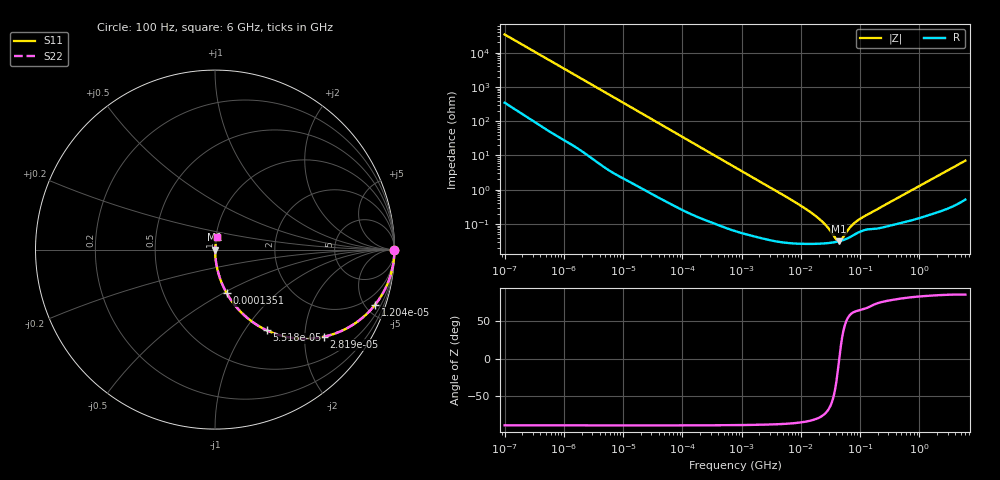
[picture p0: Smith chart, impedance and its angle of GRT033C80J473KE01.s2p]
!Murata Part Number: GRT033C80J473KE01
!These Parameters are Measured in Series Mode Connection
!Data Generated on Jun 19, 2026
!  o--ll--o
!Port1  Port2
!  o------o
!Operation Temp=25[degC], DC Bias Voltage=0[V]
!Freq. Start=100[Hz] Stop=6[GHz] 401[Steps]
# Hz S RI R 50
!Freq.(Hz) S11(Real) S11(Imag) S21(Real) S21(Imag) S12(Real) S12(Imag) S22(Real) S22(Imag)
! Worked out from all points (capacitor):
!   401 points, 100 Hz to 6 GHz, reference 50 ohm
!   read as one part in series: C = 46.6 nF near 109 Hz
!   lowest |Z| = 31.4 mohm at 43.57 MHz (marker M1)
!   series resonance near 44.57 MHz, so ESL is about 270 pH
!   S11 on the Smith chart (normalised r, x): 100 Hz: open; 12.04 kHz: 1.04, -5.79; 28.19 kHz: 1.02, -2.48; 55.18 kHz: 1.01, -1.27; 135.1 kHz: 1.00, -0.52; 6 GHz: 1.01, +0.14
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100  1 -0.00294  3.87e-05 0.00294  3.87e-05 0.00294  1 -0.00294
2008  0.9962 -0.0577  0.00379 0.0577  0.00379 0.0577  0.9962 -0.0577
5143  0.9777 -0.1444  0.0223 0.1444  0.0223 0.1444  0.9777 -0.1444
12041  0.892 -0.3073  0.108 0.3073  0.108 0.3073  0.892 -0.3073
18016  0.7884 -0.4053  0.2116 0.4053  0.2116 0.4053  0.7884 -0.4053
28191  0.6058 -0.4854  0.3942 0.4854  0.3942 0.4854  0.6058 -0.4854
40335  0.4306 -0.4918  0.5694 0.4918  0.5694 0.4918  0.4306 -0.4918
55182  0.2892 -0.45  0.7108 0.45  0.7108 0.45  0.2892 -0.45
86348  0.1439 -0.3475  0.8561 0.3475  0.8561 0.3475  0.1439 -0.3475
135116  0.0652 -0.2431  0.9348 0.2431  0.9348 0.2431  0.0652 -0.2431
302498  0.0145 -0.115  0.9855 0.115  0.9855 0.115  0.0145 -0.115
774597  0.00271 -0.0457  0.9973 0.0457  0.9973 0.0457  0.00271 -0.0457
6353432  0.000308 -0.00554  0.9997 0.00554  0.9997 0.00554  0.000308 -0.00554
1.555665e7  0.000267 -0.00203  0.9997 0.00203  0.9997 0.00203  0.000267 -0.00203
2.434276e7  0.000272 -0.00103  0.9997 0.00103  0.9997 0.00103  0.000272 -0.00103
3.983537e7  0.000302 -0.00018  0.9997 0.00018  0.9997 0.00018  0.000302 -0.00018
4.35672e7  0.000312 -3.6e-05  0.9997 3.6e-05  0.9997 3.6e-05  0.000312 -3.6e-05
4.764863e7  0.000325 0.000108  0.9997 -0.000108  0.9997 -0.000108  0.000325 0.000108
6.817316e7  0.000417 0.000689  0.9996 -0.000689  0.9996 -0.000689  0.000417 0.000689
8.918374e7  0.000544 0.00111  0.9995 -0.00111  0.9995 -0.00111  0.000544 0.00111
3.124326e8  0.000901 0.00415  0.9991 -0.00415  0.9991 -0.00415  0.000901 0.00415
6e9  0.01 0.0696  0.99 -0.0696  0.99 -0.0696  0.01 0.0696
